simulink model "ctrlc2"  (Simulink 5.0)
settings: Solver=ode15s  StartTime=0.0  StopTime=0.25  MaxStep=1e-4  RelTol=1e-3
InitFcn:
  | warning off
libraries: simulink_extras x1

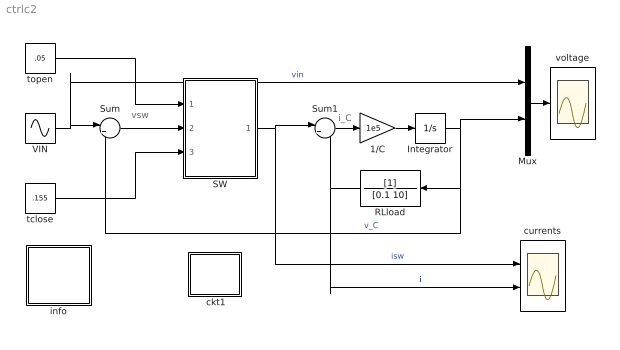
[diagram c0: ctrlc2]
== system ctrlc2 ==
  note: vsw
  note: i_C
  " ckt1" : Subsystem
  1/C : Gain  Gain=1e5
  Integrator : Integrator
  Mux : Mux  Inputs=2
  RLload : TransferFcn  Orientation=left  Denominator=[0.1 10]
  SW : Subsystem
  Sum : Sum  Inputs=|+-
  Sum1 : Sum  Inputs=|+-
  VIN : Sin  Amplitude=120*sqrt(2)  Frequency=2*pi*60  SampleTime=0
  currents : Scope  NumInputPorts=2
  info : Subsystem
  tclose : Constant  Value=.155
  topen : Constant  Value=.05
  voltage : Scope
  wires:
  VIN/1 -> Sum/1, Mux/1  "vin"
  Sum/1 -> SW/2(vsw)
  Sum1/1 -> 1/C/1
  1/C/1 -> Integrator/1
  Integrator/1 -> RLload/1, Sum/2, Mux/2  "v_C"
  RLload/1 -> Sum1/2, currents/2  "i_L"
  topen/1 -> SW/1(open)
  tclose/1 -> SW/3(close)
  SW/1(isw) -> Sum1/1, currents/1  "isw"
  Mux/1 -> voltage/1

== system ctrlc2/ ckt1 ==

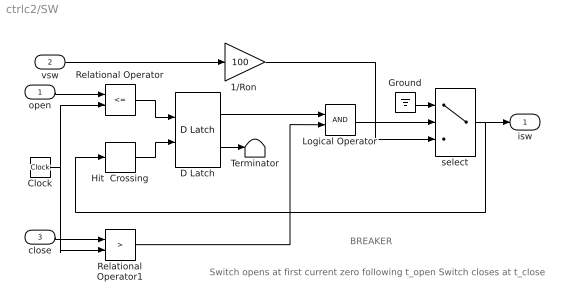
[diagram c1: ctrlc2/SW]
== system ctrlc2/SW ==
  note: Switch opens at first current zero following t_open Switch closes at t_close
  note: BREAKER
  open : Inport
  vsw : Inport  Port=2
  close : Inport  Port=3
  "1/Ron " : Gain  Gain=100
  Clock : Clock
  D Latch : simulink_extras/Flip Flops/D Latch
  Ground : Ground
  Hit  Crossing : HitCross
  Logical Operator : Logic
  Relational Operator : RelationalOperator  Operator=<=
  Relational Operator1 : RelationalOperator  Operator=>
  Terminator : Terminator
  select : Switch  Threshold=0.5
  isw : Outport
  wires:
  D Latch/2 -> Terminator/1
  Hit  Crossing/1 -> D Latch/2
  Ground/1 -> select/1
  Logical Operator/1 -> select/2
  open/1 -> Relational Operator/1
  Relational Operator1/1 -> Logical Operator/2
  close/1 -> Relational Operator1/1
  select/1 -> isw/1, Hit  Crossing/1
  vsw/1 -> "1/Ron "/1
  "1/Ron "/1 -> select/3
  Clock/1 -> Relational Operator/2, Relational Operator1/2
  Relational Operator/1 -> D Latch/1
  D Latch/1 -> Logical Operator/1

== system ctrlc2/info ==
  note: RLC switched circuit
  note: A series RL load in parallel with a capacitor operates under sinusoidal voltage excitation for a specified length of time "topen" when, at the first subsequent current zero, a circuit breaker connected between the source and the load suddenly opens to reclose later at a specified time "tclose". The circuit breaker is simulated by means of a switch block activated by a D latch flipflop block which determines a zero-crossing immediately following the commanded time "topen". (To simulate the breaker opening at "topen" under current chopping, simply delete the portion involving the latch). Reclosure takes place at time "tclose". The source current isw as well as the load current iL and the capacitor voltage vC are exhibited as functions of time.
